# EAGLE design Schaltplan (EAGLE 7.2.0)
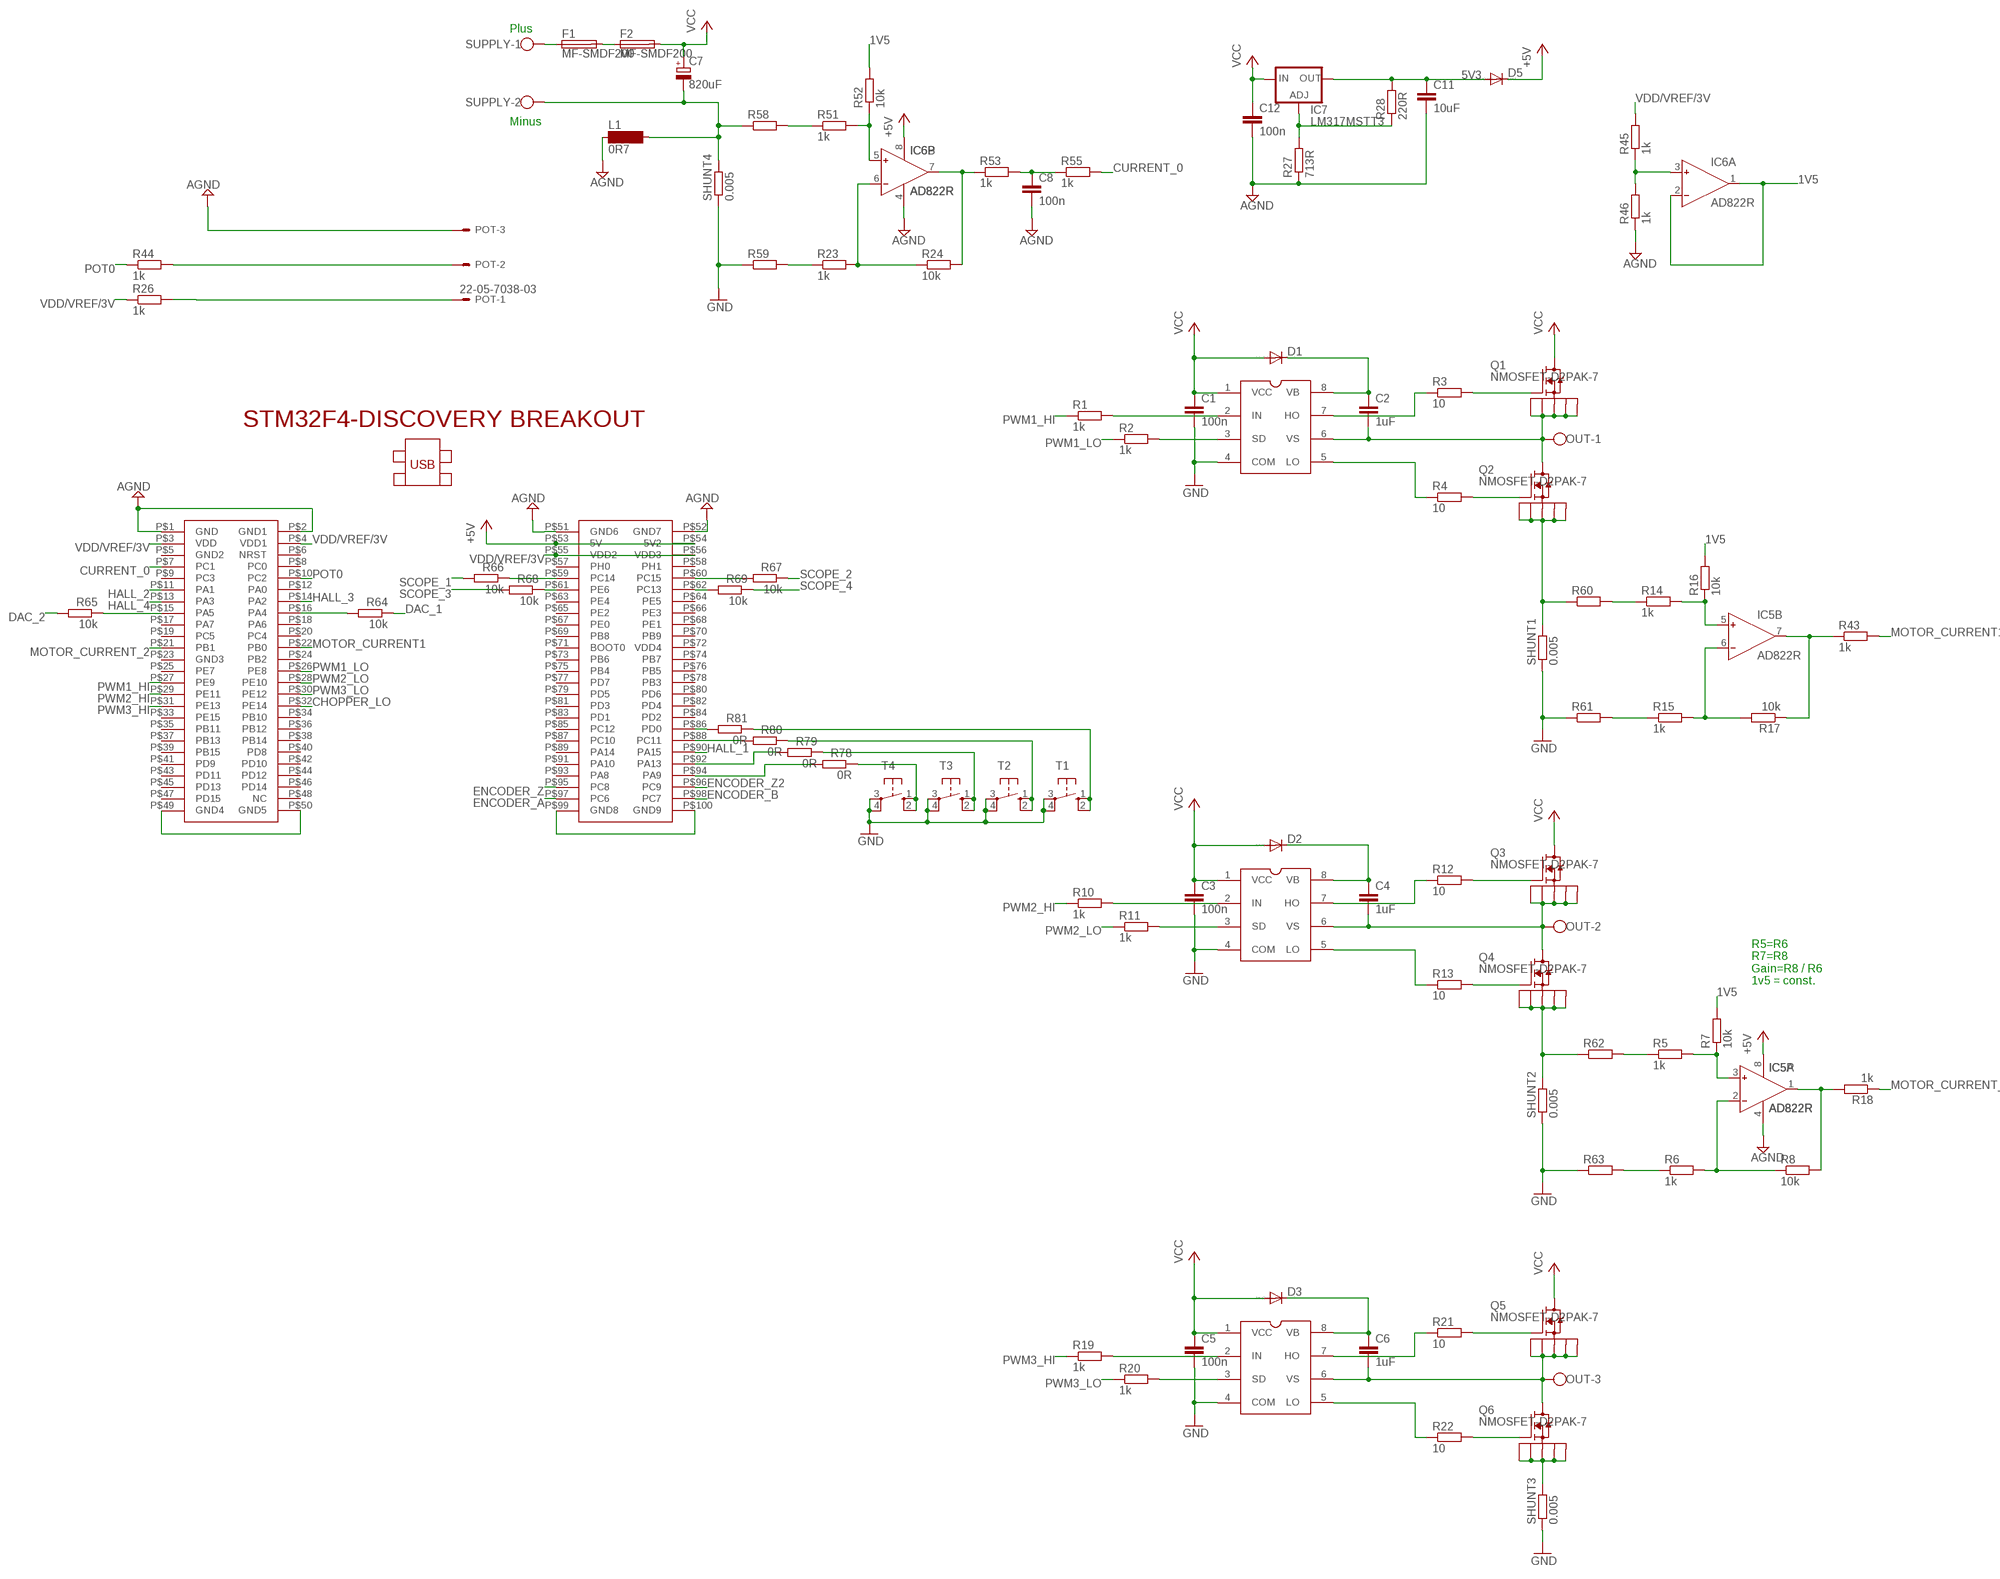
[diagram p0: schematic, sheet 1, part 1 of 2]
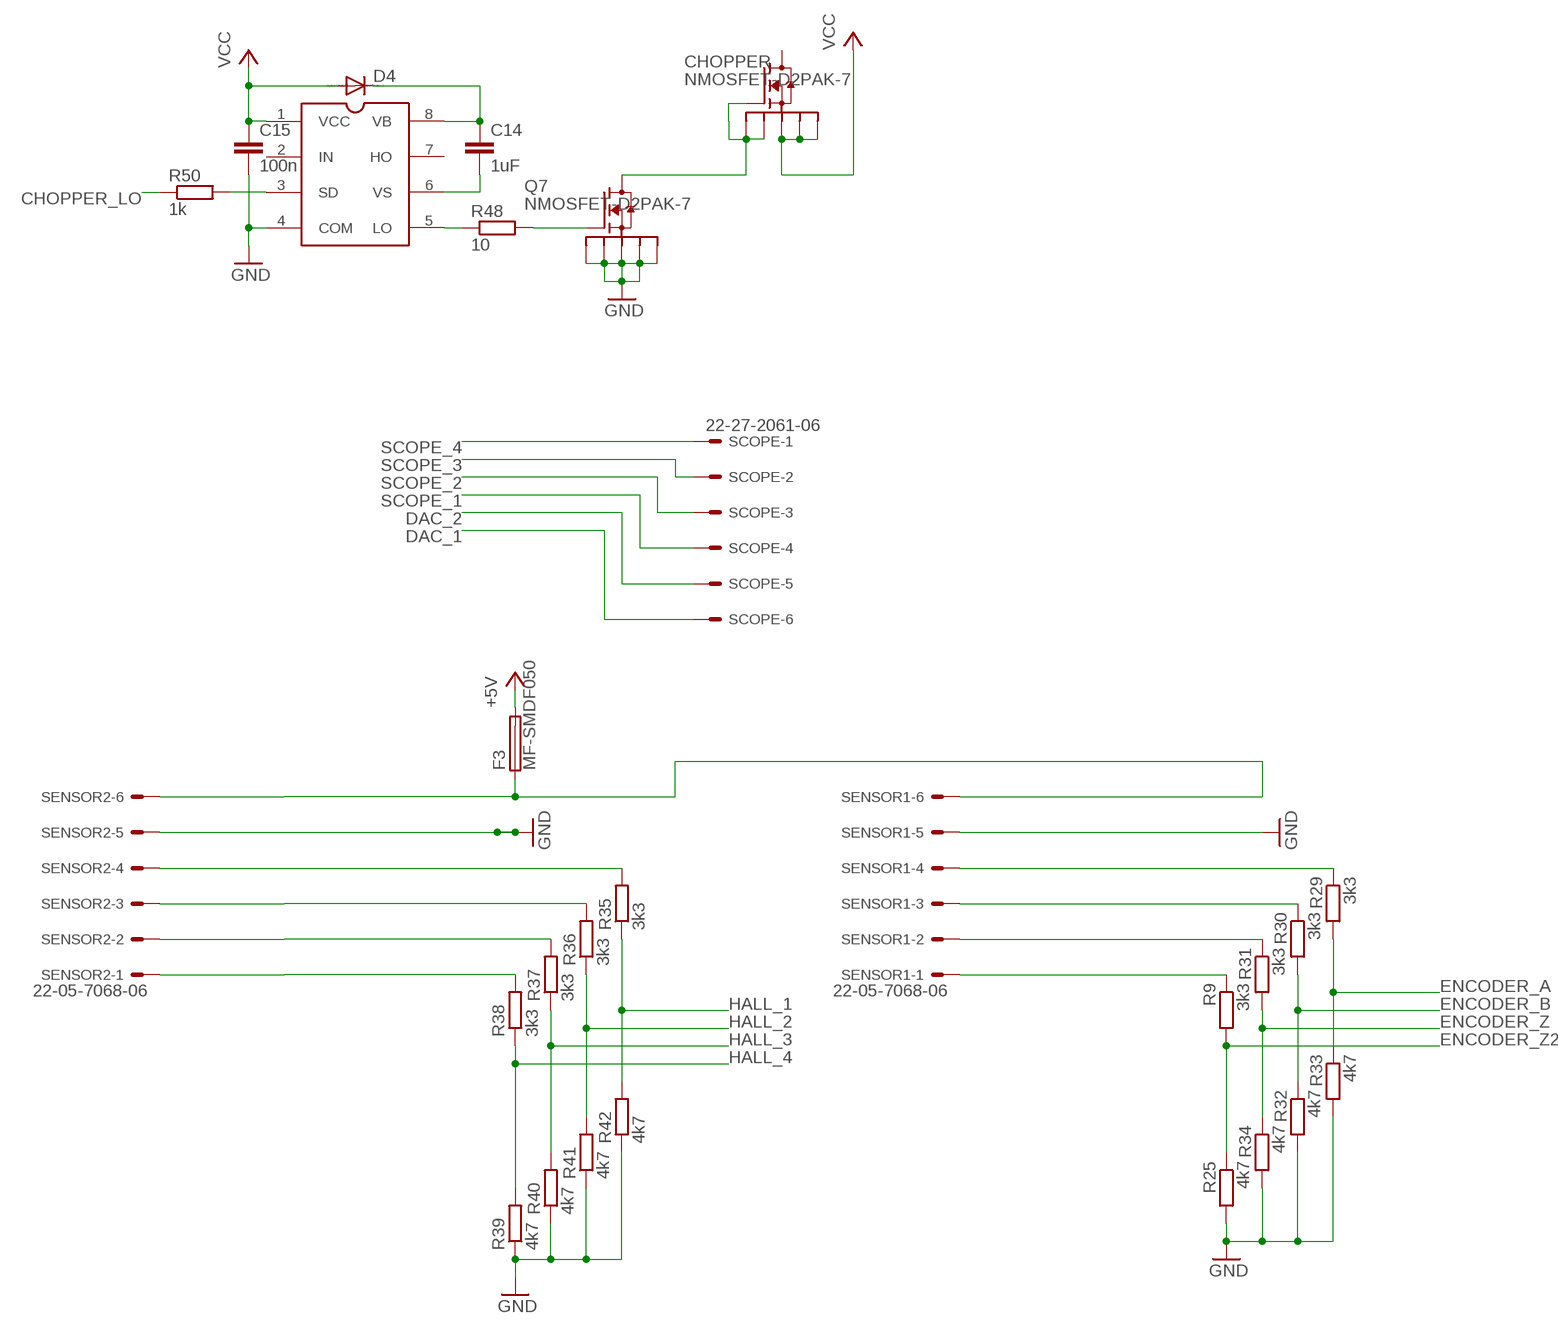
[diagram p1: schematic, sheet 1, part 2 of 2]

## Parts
C1  100n  C-EUC0805K  [C0805K]
C2  1uF  C-EUC0805K  [C0805K]
C3  100n  C-EUC0805K  [C0805K]
C4  1uF  C-EUC0805K  [C0805K]
C5  100n  C-EUC0805K  [C0805K]
C6  1uF  C-EUC0805K  [C0805K]
C7  820uF  CPOL-EUE7.5-18  [E7,5-18]
C8  100n  C-EUC0805K  [C0805K]
C11  10uF  C-EUC0805K  [C0805K]
C12  100n  C-EUC0805K  [C0805K]
C14  1uF  C-EUC0805K  [C0805K]
C15  100n  C-EUC0805K  [C0805K]
CHOPPER  NMOSFET-D2PAK-7  [D2PAK-7]
D1  DIODE-DO214AC  [DO214AC]
D2  DIODE-DO214AC  [DO214AC]
D3  DIODE-DO214AC  [DO214AC]
D4  DIODE-DO214AC  [DO214AC]
D5  DIODE-DO214AC  [DO214AC]
F1  MF-SMDF200  [MF-SMDF050]
F2  MF-SMDF200  [MF-SMDF050]
F3  MF-SMDF050  [MF-SMDF050]
IC1  IR2104S  [IR2104S]
IC2  IR2104S  [IR2104S]
IC3  IR2104S  [IR2104S]
IC4  IR2104S  [IR2104S]
IC5  AD822R  [SO8]
IC6  AD822R  [SO8]
IC7  LM317MSTT3  [SOT223]
L1  0R7  SM-1206  [SM-1206]
OUT  W237-103  [W237-103]
POT  22-05-7038-03  [7395-03]
Q1  NMOSFET-D2PAK-7  [D2PAK-7]
Q2  NMOSFET-D2PAK-7  [D2PAK-7]
Q3  NMOSFET-D2PAK-7  [D2PAK-7]
Q4  NMOSFET-D2PAK-7  [D2PAK-7]
Q5  NMOSFET-D2PAK-7  [D2PAK-7]
Q6  NMOSFET-D2PAK-7  [D2PAK-7]
Q7  NMOSFET-D2PAK-7  [D2PAK-7]
R1  1k  R-EU_M0805  [M0805]
R2  1k  R-EU_M0805  [M0805]
R3  10  R-EU_M0805  [M0805]
R4  10  R-EU_M0805  [M0805]
R5  1k  R-EU_M0805  [M0805]
R6  1k  R-EU_M0805  [M0805]
R7  10k  R-EU_M0805  [M0805]
R8  10k  R-EU_M0805  [M0805]
R9  3k3  R-EU_M0805  [M0805]
R10  1k  R-EU_M0805  [M0805]
R11  1k  R-EU_M0805  [M0805]
R12  10  R-EU_M0805  [M0805]
R13  10  R-EU_M0805  [M0805]
R14  1k  R-EU_M0805  [M0805]
R15  1k  R-EU_M0805  [M0805]
R16  10k  R-EU_M0805  [M0805]
R17  10k  R-EU_M0805  [M0805]
R18  1k  R-EU_M0805  [M0805]
R19  1k  R-EU_M0805  [M0805]
R20  1k  R-EU_M0805  [M0805]
R21  10  R-EU_M0805  [M0805]
R22  10  R-EU_M0805  [M0805]
R23  1k  R-EU_M0805  [M0805]
R24  10k  R-EU_M0805  [M0805]
R25  4k7  R-EU_M0805  [M0805]
R26  1k  R-EU_M0805  [M0805]
R27  713R  R-EU_M0805  [M0805]
R28  220R  R-EU_M0805  [M0805]
R29  3k3  R-EU_M0805  [M0805]
R30  3k3  R-EU_M0805  [M0805]
R31  3k3  R-EU_M0805  [M0805]
R32  4k7  R-EU_M0805  [M0805]
R33  4k7  R-EU_M0805  [M0805]
R34  4k7  R-EU_M0805  [M0805]
R35  3k3  R-EU_M0805  [M0805]
R36  3k3  R-EU_M0805  [M0805]
R37  3k3  R-EU_M0805  [M0805]
R38  3k3  R-EU_M0805  [M0805]
R39  4k7  R-EU_M0805  [M0805]
R40  4k7  R-EU_M0805  [M0805]
R41  4k7  R-EU_M0805  [M0805]
R42  4k7  R-EU_M0805  [M0805]
R43  1k  R-EU_M0805  [M0805]
R44  1k  R-EU_M0805  [M0805]
R45  1k  R-EU_M0805  [M0805]
R46  1k  R-EU_M0805  [M0805]
R48  10  R-EU_M0805  [M0805]
R50  1k  R-EU_M0805  [M0805]
R51  1k  R-EU_M0805  [M0805]
R52  10k  R-EU_M0805  [M0805]
R53  1k  R-EU_M0805  [M0805]
R55  1k  R-EU_M0805  [M0805]
R58  R-EU_M0805  [M0805]
R59  R-EU_M0805  [M0805]
R60  R-EU_M0805  [M0805]
R61  R-EU_M0805  [M0805]
R62  R-EU_M0805  [M0805]
R63  R-EU_M0805  [M0805]
R64  10k  R-EU_M0805  [M0805]
R65  10k  R-EU_M0805  [M0805]
R66  10k  R-EU_M0805  [M0805]
R67  10k  R-EU_M0805  [M0805]
R68  10k  R-EU_M0805  [M0805]
R69  10k  R-EU_M0805  [M0805]
R78  0R  R-EU_M0805  [M0805]
R79  0R  R-EU_M0805  [M0805]
R80  0R  R-EU_M0805  [M0805]
R81  0R  R-EU_M0805  [M0805]
SCOPE  22-27-2061-06  [6410-06]
SENSOR1  22-05-7068-06  [7395-06]
SENSOR2  22-05-7068-06  [7395-06]
SHUNT1  0.005  R-EU_R2512  [R2512]
SHUNT2  0.005  R-EU_R2512  [R2512]
SHUNT3  0.005  R-EU_R2512  [R2512]
SHUNT4  0.005  R-EU_R2512  [R2512]
SUPPLY  W237-102  [W237-102]
T1  10-XX  [B3F-10XX]
T2  10-XX  [B3F-10XX]
T3  10-XX  [B3F-10XX]
T4  10-XX  [B3F-10XX]
U$1  STM32F4-DISCOVERY  [STM32F4-DISCOVERY]

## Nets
1: C2.2 IC1.6(VS) OUT.1 Q1.S1 Q1.S2 Q1.S3 Q1.S4 Q1.S5 Q2.D
1V5: IC6.1(A:OUT) IC6.2(A:IN-) R7.2 R16.2 R52.2
2: C4.2 IC2.6(VS) OUT.2 Q3.S1 Q3.S2 Q3.S3 Q3.S4 Q3.S5 Q4.D
3 [power]: C6.2 IC3.6(VS) OUT.3 Q5.S1 Q5.S2 Q5.S3 Q5.S4 Q5.S5 Q6.D
5V3: C11.1 D5.A IC7.4(OUT) R28.2
+5V: D5.C F3.2 IC5.8(P:V+) IC6.8(P:V+) U$1.P$53(5V) U$1.P$54(5V2)
AGND: C8.2 C11.2 C12.2 IC5.4(P:V-) IC6.4(P:V-) L1.1 POT.3 R27.1 R46.1 U$1.P$1(GND) U$1.P$2(GND1) U$1.P$51(GND6) U$1.P$52(GND7)
CHOPPER_LO: R50.1 U$1.P$32(PE14)
CURRENT_0: R55.2 U$1.P$7(PC1)
DAC_1: R64.1 SCOPE.6
DAC_2: R65.2 SCOPE.5
ENCODER_A: R29.2 R33.1 U$1.P$97(PC6)
ENCODER_B: R30.2 R32.1 U$1.P$98(PC7)
ENCODER_Z: R31.2 R34.1 U$1.P$95(PC8)
ENCODER_Z2: R9.2 R25.1 U$1.P$96(PC9)
GND [power]: C1.2 C3.2 C5.2 C15.2 IC1.4(COM) IC2.4(COM) IC3.4(COM) IC4.4(COM) Q7.S1 Q7.S2 Q7.S3 Q7.S4 Q7.S5 R25.2 R32.2 R33.2 R34.2 R39.1 R40.1 R41.1 R42.1 R59.1 R61.1 R63.1 SENSOR1.5 SENSOR2.5 SHUNT1.1 SHUNT2.1 SHUNT3.1 SHUNT4.1 T1.3(P) T1.4(P1) T2.3(P) T2.4(P1) T3.3(P) T3.4(P1) T4.3(P) T4.4(P1)
HALL_1: R35.1 R42.2 U$1.P$90(PA15)
HALL_2: R36.1 R41.2 U$1.P$11(PA1)
HALL_3: R37.1 R40.2 U$1.P$14(PA2)
HALL_4: R38.1 R39.2 U$1.P$13(PA3)
MOTOR_CURRENT1: R43.2 U$1.P$22(PB0)
MOTOR_CURRENT_2: R18.1 U$1.P$21(PB1)
N$1: IC1.7(HO) R3.1
N$2: Q1.G R3.2
N$3: Q2.G R4.2
N$4: IC1.5(LO) R4.1
N$5: C2.1 D1.C IC1.8(VB)
N$6: IC2.7(HO) R12.1
N$7: IC5.2(A:IN-) R6.2 R8.1
N$8: IC1.2(IN) R1.2
N$9: IC1.3(SD) R2.2
N$10: Q3.G R12.2
N$11: Q2.S1 Q2.S2 Q2.S3 Q2.S4 Q2.S5 R60.1 SHUNT1.2
N$12: IC5.3(A:IN+) R5.2 R7.1
N$13: IC5.1(A:OUT) R8.2 R18.2
N$14: Q4.G R13.2
N$15: IC2.5(LO) R13.1
N$16: C4.1 D2.C IC2.8(VB)
N$17: IC2.2(IN) R10.2
N$18: IC2.3(SD) R11.2
N$19: Q4.S1 Q4.S2 Q4.S3 Q4.S4 Q4.S5 R62.1 SHUNT2.2
N$20: IC5.5(B:IN+) R14.2 R16.1
N$21: IC5.6(B:IN-) R15.2 R17.2
N$22: IC5.7(B:OUT) R17.1 R43.1
N$23: IC3.7(HO) R21.1
N$24: Q5.G R21.2
N$25: Q6.G R22.2
N$26: IC3.5(LO) R22.1
N$27: C6.1 D3.C IC3.8(VB)
N$28: IC3.2(IN) R19.2
N$29: IC3.3(SD) R20.2
N$30: R23.1 R59.2
N$31: F3.1 SENSOR1.6 SENSOR2.6
N$32: IC6.3(A:IN+) R45.1 R46.2
N$33: IC7.1(ADJ) R27.2 R28.1
N$34: R29.1 SENSOR1.4
N$35: R30.1 SENSOR1.3
N$36: C8.1 R53.2 R55.1
N$37: R31.1 SENSOR1.2
N$38: R64.2 U$1.P$16(PA4)
N$39: R65.1 U$1.P$15(PA5)
N$40: R79.2 U$1.P$92(PA13)
N$41: R9.1 SENSOR1.1
N$42: R35.2 SENSOR2.4
N$43: R36.2 SENSOR2.3
N$44: R37.2 SENSOR2.2
N$45: R38.2 SENSOR2.1
N$46: R66.1 U$1.P$59(PC14)
N$47: R68.1 U$1.P$61(PE6)
N$48: R69.2 U$1.P$62(PC13)
N$49: R67.2 U$1.P$60(PC15)
N$50: POT.1 R26.2
N$51: R80.2 U$1.P$88(PC11)
N$52: R81.2 U$1.P$86(PD0)
N$53: CHOPPER.G CHOPPER.S1 CHOPPER.S2 Q7.D
N$54: R51.1 R58.2
N$55: R78.1 T4.1(S) T4.2(S1)
N$56: R5.1 R62.2
N$57: POT.2 R44.2
N$58: R78.2 U$1.P$94(PA9)
N$59: R79.1 T3.1(S) T3.2(S1)
N$62 [power]: F1.1 SUPPLY.1
N$63 [power]: C7.- L1.2 R58.1 SHUNT4.2 SUPPLY.2
N$64: R80.1 T2.1(S) T2.2(S1)
N$68: R6.1 R63.2
N$71: Q7.G R48.2
N$72: IC6.6(B:IN-) R23.2 R24.1
N$73: C14.1 D4.C IC4.8(VB)
N$74: C14.2 IC4.6(VS)
N$75: IC4.5(LO) R48.1
N$77: IC4.3(SD) R50.2
N$79: IC6.7(B:OUT) R24.2 R53.1
N$80: IC6.5(B:IN+) R51.2 R52.1
N$83: F1.2 F2.1
N$84: R81.1 T1.1(S) T1.2(S1)
N$85: R14.1 R60.2
N$86: R15.1 R61.2
N$89: Q6.S1 Q6.S2 Q6.S3 Q6.S4 Q6.S5 SHUNT3.2
N$91: U$1.P$99(GND8) U$1.P$100(GND9)
N$92: U$1.P$49(GND4) U$1.P$50(GND5)
POT0: R44.1 U$1.P$10(PC2)
PWM1_HI: R1.1 U$1.P$27(PE9)
PWM1_LO: R2.1 U$1.P$26(PE8)
PWM2_HI: R10.1 U$1.P$29(PE11)
PWM2_LO: R11.1 U$1.P$28(PE10)
PWM3_HI: R19.1 U$1.P$31(PE13)
PWM3_LO: R20.1 U$1.P$30(PE12)
SCOPE_1: R66.2 SCOPE.4
SCOPE_2: R67.1 SCOPE.3
SCOPE_3: R68.2 SCOPE.2
SCOPE_4: R69.1 SCOPE.1
VCC [power]: C1.1 C3.1 C5.1 C7.+ C12.1 C15.1 CHOPPER.S3 CHOPPER.S4 CHOPPER.S5 D1.A D2.A D3.A D4.A F2.2 IC1.1(VCC) IC2.1(VCC) IC3.1(VCC) IC4.1(VCC) IC7.3(IN) Q1.D Q3.D Q5.D
VDD/VREF/3V: R26.1 R45.2 U$1.P$3(VDD) U$1.P$4(VDD1) U$1.P$55(VDD2) U$1.P$56(VDD3)
Unconnected: CHOPPER.D IC4.2(IN) IC4.7(HO) U$1.P$5(GND2) U$1.P$6(NRST) U$1.P$8(PC0) U$1.P$9(PC3) U$1.P$12(PA0) U$1.P$17(PA7) U$1.P$18(PA6) U$1.P$19(PC5) U$1.P$20(PC4) U$1.P$23(GND3) U$1.P$24(PB2) U$1.P$25(PE7) U$1.P$33(PE15) U$1.P$34(PB10) U$1.P$35(PB11) U$1.P$36(PB12) U$1.P$37(PB13) U$1.P$38(PB14) U$1.P$39(PB15) U$1.P$40(PD8) U$1.P$41(PD9) U$1.P$42(PD10) U$1.P$43(PD11) U$1.P$44(PD12) U$1.P$45(PD13) U$1.P$46(PD14) U$1.P$47(PD15) U$1.P$48(NC) U$1.P$57(PH0) U$1.P$58(PH1) U$1.P$63(PE4) U$1.P$64(PE5) U$1.P$65(PE2) U$1.P$66(PE3) U$1.P$67(PE0) U$1.P$68(PE1) U$1.P$69(PB8) U$1.P$70(PB9) U$1.P$71(BOOT0) U$1.P$72(VDD4) U$1.P$73(PB6) U$1.P$74(PB7) U$1.P$75(PB4) U$1.P$76(PB5) U$1.P$77(PD7) U$1.P$78(PB3) U$1.P$79(PD5) U$1.P$80(PD6) U$1.P$81(PD3) U$1.P$82(PD4) U$1.P$83(PD1) U$1.P$84(PD2) U$1.P$85(PC12) U$1.P$87(PC10) U$1.P$89(PA14) U$1.P$91(PA10) U$1.P$93(PA8)

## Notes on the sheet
- Plus
- Minus
- R5=R6
  R7=R8
  Gain=R8 / R6
  1v5 = const.

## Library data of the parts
C1-C6 C8 C11 C12 C14 C15 = rcl:C-EU: CAPACITOR, European symbol
C7 = rcl:CPOL-EU: POLARIZED CAPACITOR, European symbol
CHOPPER Q1-Q7 = D2PAK-7:NMOSFET-D2PAK-7
D1-D5 = diode:DIODE-: DIODE
F1-F3 = fuse:MF-SMDF: MF-SMDF Series - PRC Resettable Fuses
IC1-IC4 = ir-2104:IR2104S: Half Bridge Mosfet - IGBT driver SOIC
IC5 IC6 = analog-devices:AD822: Single-Supply, Rail-to-Rail Low Power FET-Input Op Amp Source: http://www.analog.com/static/imported-files/data_sheets/AD822.pdf; MF: ANALOG DEVICES; MPN: AD822BRZ; OC_FARNELL: 1651303
IC7 = v-reg:LM317?*: 500 mA Adjustable Output Positive Voltage Regulator Source: http://www.onsemi.co.jp .. LM317M-D.PDF
L1 = inductor-neosid:SM-1206: INDUCTOR; OC_FARNELL: unknown; OC_NEWARK: unknown
OUT = con-wago-500:W237-103: WAGO SCREW CLAMP; MPN: 237-103; OC_FARNELL: unknown; OC_NEWARK: 18M7116
POT = con-molex:22-?-03: CONNECTOR wire to board 2.54 mm (.1 inch) pitch header; OC_FARNELL: unknown; OC_NEWARK: unknown
R1-R5 R7-R46 R48 R50-R53 R55 R64-R69 R78-R81 = resistor:R-EU_: RESISTOR, European symbol
R6 R58-R63 SHUNT1-SHUNT4 = rcl:R-EU_: RESISTOR, European symbol
SCOPE SENSOR1 SENSOR2 = con-molex:22-?-06: CONNECTOR wire to board 2.54 mm (.1 inch) pitch header; OC_FARNELL: unknown; OC_NEWARK: unknown
SUPPLY = con-wago-500:W237-102: WAGO SCREW CLAMP; MPN: 237-102; OC_FARNELL: unknown; OC_NEWARK: 70K9898
T1-T4 = switch-omron:10-XX: OMRON SWITCH; MPN: B3F-1000; OC_FARNELL: 176432; OC_NEWARK: 36M3542
U$1 = STM32F4-DISCOVERY:STM32F4-DISCOVERY

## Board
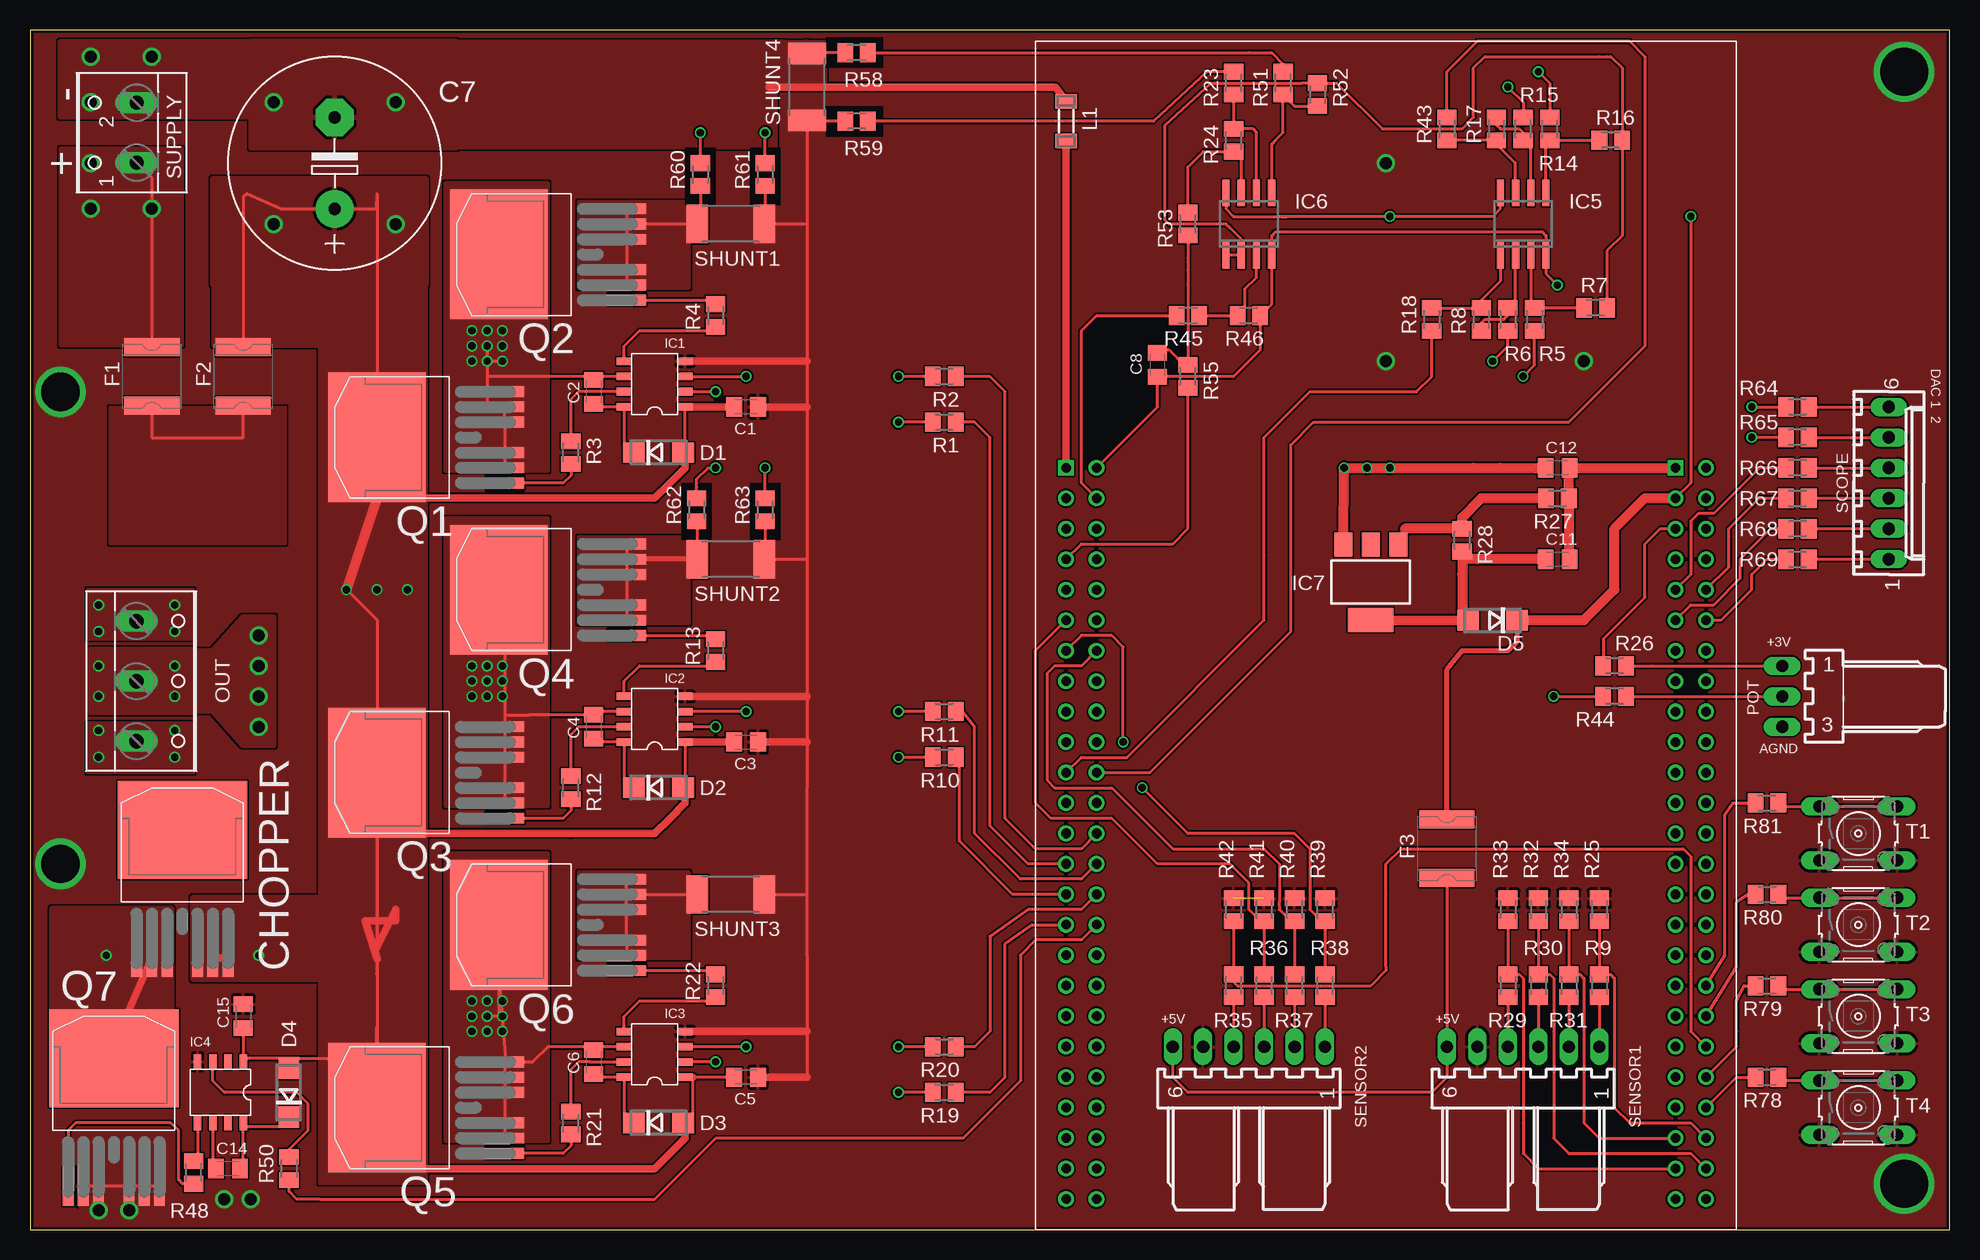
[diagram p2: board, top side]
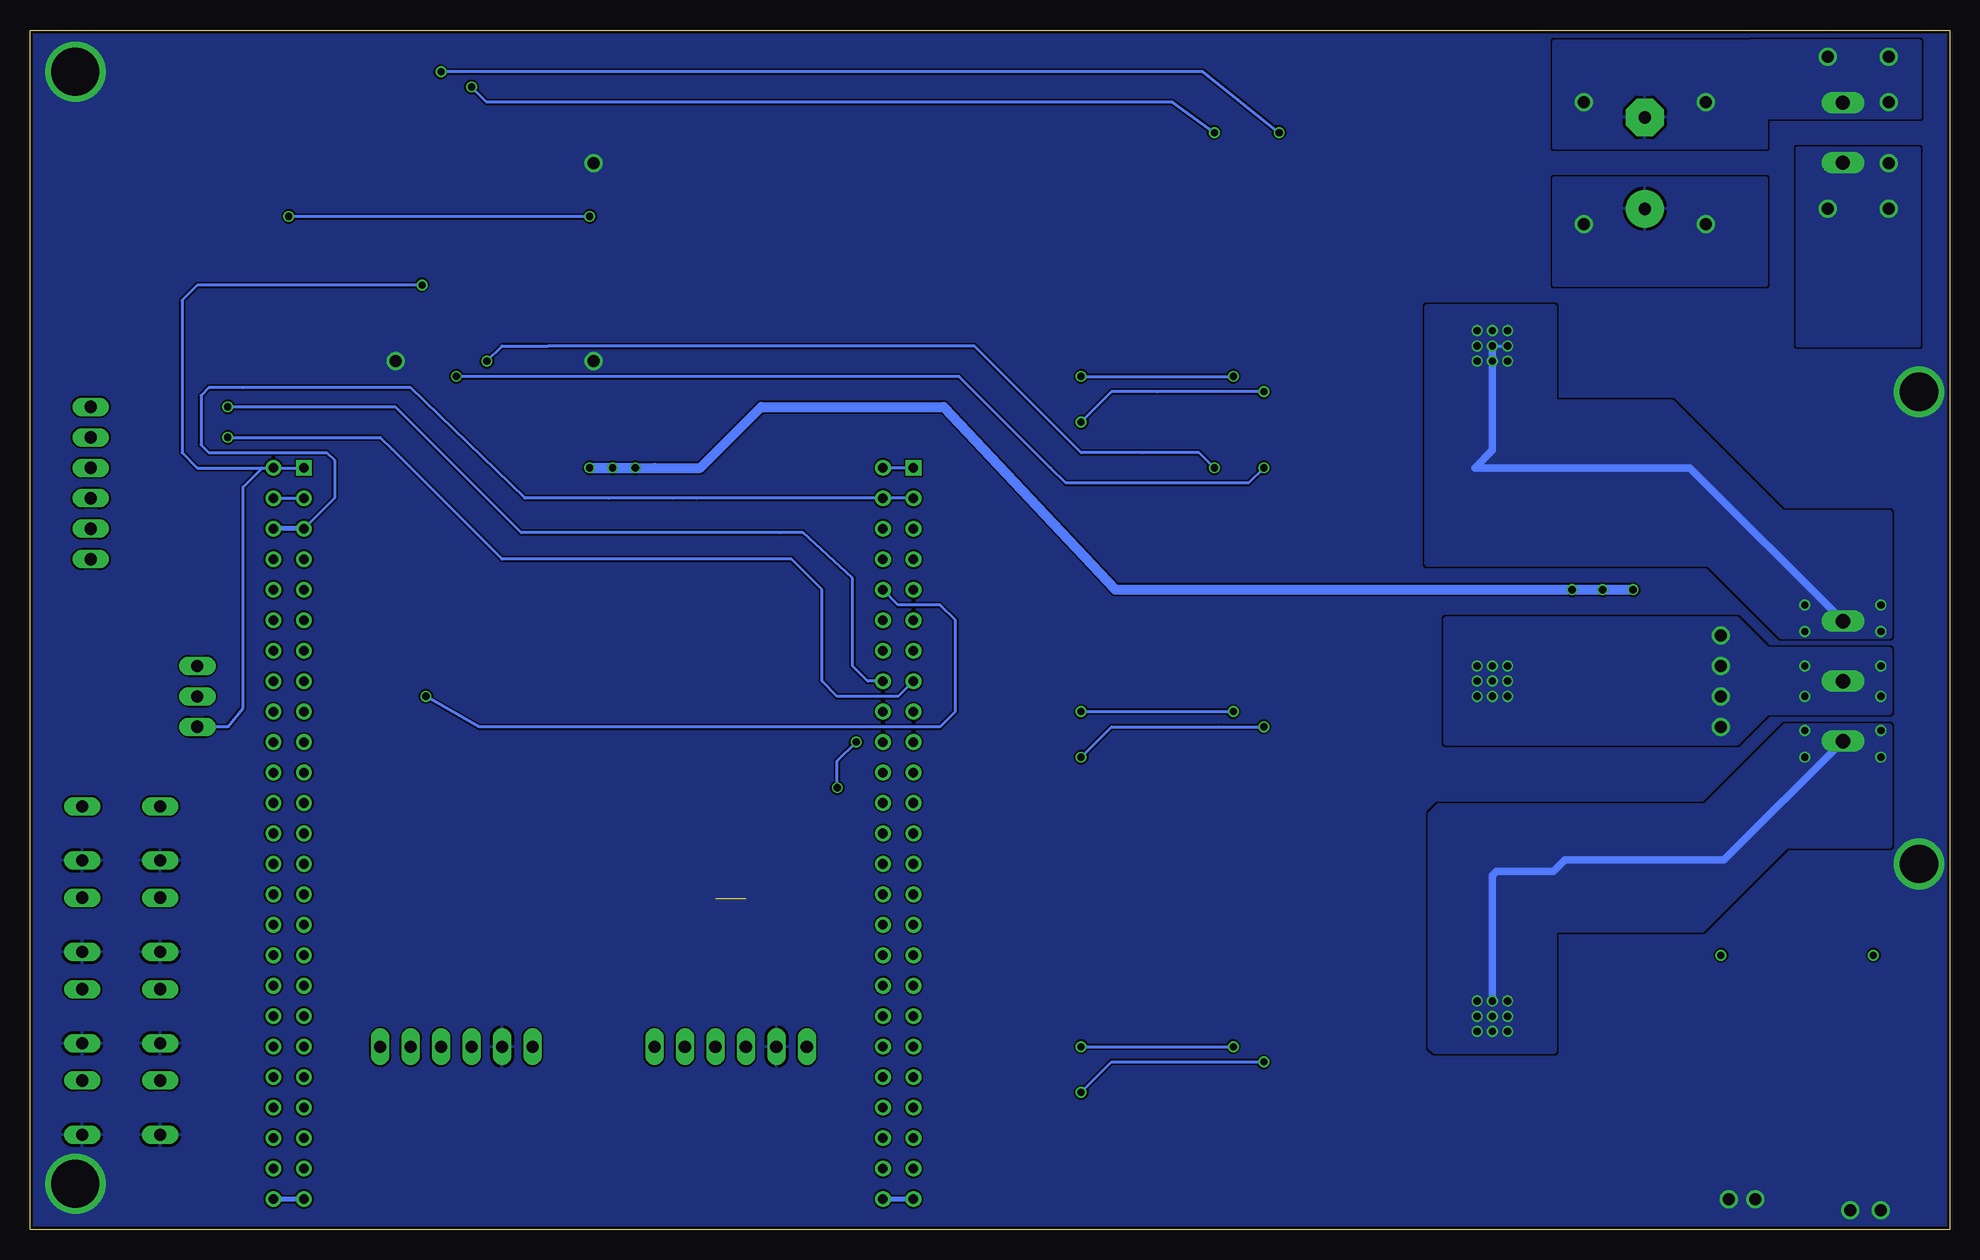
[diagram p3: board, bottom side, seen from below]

Size 160 x 100 mm. Coordinates in mm from the lower left corner, seen from the top.
Outline: 0,0 160,0 160,100 0,100 0,0
Copper layers (1*16): Top 0.035mm / dielectric 1.5mm / Bottom 0.035mm
Design rules "Elecrow_2-layer_eagle_rule": minimum track width 6mil, minimum drill 12mil, track to track 6mil, track to pad 6mil, pad to pad 6mil, via to via 6mil, smd to smd 0mil, copper to edge 10mil, drill to drill 10mil, minimum pad ring 10mil, minimum via ring 6mil, stop-mask expansion 2mil, vias tented up to drill 100mil, thermal gap 10mil

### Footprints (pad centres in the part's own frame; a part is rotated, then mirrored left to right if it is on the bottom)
C0805K = smd 1.3 x 1.6: 1 -1,0; 2 1,0
E7,5-18 = drill 1.016 pad 3.15: + -3.81,0 | drill 1.016 pad 3.15 octagon: - 3.81,0
D2PAK-7 = smd 10.8 x 8.15: D 0,4.1 | smd 0.9 x 3.2: G -3.81,-6.56; S1 -2.54,-6.56; S2 -1.27,-6.56; S3 1.27,-6.56; S4 2.54,-6.56; S5 3.81,-6.56
DO214AC = smd 1.8 x 1.7: A 2.05,0; C -2.05,0
MF-SMDF050 = smd 1.5 x 4.6: 1 -2.45,0; 2 2.45,0
IR2104S = smd 1.27 x 0.635: 1 0,3.81; 2 0,2.54; 3 0,1.27; 4 0,0; 5 5.08,0; 6 5.08,1.27; 7 5.08,2.54; 8 5.08,3.81
SO8 = smd 0.6 x 2.2: 1 -1.905,-2.6; 2 -0.635,-2.6; 3 0.635,-2.6; 4 1.905,-2.6; 5 1.905,2.6; 6 0.635,2.6; 7 -0.635,2.6; 8 -1.905,2.6
SOT223 = smd 1.5 x 2: 1 -2.3,-3.15; 2 0,-3.15; 3 2.3,-3.15 | smd 3.8 x 2: 4 0,3.15
SM-1206 = smd 1.2 x 1.8: 1 -1.65,0; 2 1.65,0
W237-103 = drill 1.194 long: 1 -5,-1.29; 2 0,-1.29; 3 5,-1.29
7395-03 = drill 1.016 long: 1 2.54,0; 2 0,0; 3 -2.54,0
M0805 = smd 1.3 x 1.6: 1 -0.95,0; 2 0.95,0
6410-06 = drill 1.016 long: 1 6.35,0; 2 3.81,0; 3 1.27,0; 4 -1.27,0; 5 -3.81,0; 6 -6.35,0
7395-06 = drill 1.016 long: 1 6.35,0; 2 3.81,0; 3 1.27,0; 4 -1.27,0; 5 -3.81,0; 6 -6.35,0
R2512 = smd 1.8 x 3.2: 1 -2.8,0; 2 2.8,0
W237-102 = drill 1.194 long: 1 -2.5,-1.27; 2 2.5,-1.27
B3F-10XX = drill 1.016 long: 1 -3.251,2.261; 2 3.251,2.261; 3 -3.251,-2.261; 4 3.251,-2.261
STM32F4-DISCOVERY = drill 0.8 square: P$1 -27.94,30.48; P$51 22.86,30.48 | drill 0.8: P$2 -25.4,30.48; P$3 -27.94,27.94; P$4 -25.4,27.94; P$5 -27.94,25.4; P$6 -25.4,25.4; P$7 -27.94,22.86; P$8 -25.4,22.86; P$9 -27.94,20.32; P$10 -25.4,20.32; P$11 -27.94,17.78; P$12 -25.4,17.78; P$13 -27.94,15.24; P$14 -25.4,15.24; P$15 -27.94,12.7; P$16 -25.4,12.7; P$17 -27.94,10.16; P$18 -25.4,10.16; P$19 -27.94,7.62; P$20 -25.4,7.62; P$21 -27.94,5.08; P$22 -25.4,5.08; P$23 -27.94,2.54; P$24 -25.4,2.54; P$25 -27.94,0; P$26 -25.4,0; P$27 -27.94,-2.54; P$28 -25.4,-2.54; P$29 -27.94,-5.08; P$30 -25.4,-5.08; P$31 -27.94,-7.62; P$32 -25.4,-7.62; P$33 -27.94,-10.16; P$34 -25.4,-10.16; P$35 -27.94,-12.7; P$36 -25.4,-12.7; P$37 -27.94,-15.24; P$38 -25.4,-15.24; P$39 -27.94,-17.78; P$40 -25.4,-17.78; P$41 -27.94,-20.32; P$42 -25.4,-20.32; P$43 -27.94,-22.86; P$44 -25.4,-22.86; P$45 -27.94,-25.4; P$46 -25.4,-25.4; P$47 -27.94,-27.94; P$48 -25.4,-27.94; P$49 -27.94,-30.48; P$50 -25.4,-30.48; P$52 25.4,30.48; P$53 22.86,27.94; P$54 25.4,27.94; P$55 22.86,25.4; P$56 25.4,25.4; P$57 22.86,22.86; P$58 25.4,22.86; P$59 22.86,20.32; P$60 25.4,20.32; P$61 22.86,17.78; P$62 25.4,17.78; P$63 22.86,15.24; P$64 25.4,15.24; P$65 22.86,12.7; P$66 25.4,12.7; P$67 22.86,10.16; P$68 25.4,10.16; P$69 22.86,7.62; P$70 25.4,7.62; P$71 22.86,5.08; P$72 25.4,5.08; P$73 22.86,2.54; P$74 25.4,2.54; P$75 22.86,0; P$76 25.4,0; P$77 22.86,-2.54; P$78 25.4,-2.54; P$79 22.86,-5.08; P$80 25.4,-5.08; P$81 22.86,-7.62; P$82 25.4,-7.62; P$83 22.86,-10.16; P$84 25.4,-10.16; P$85 22.86,-12.7; P$86 25.4,-12.7; P$87 22.86,-15.24; P$88 25.4,-15.24; P$89 22.86,-17.78; P$90 25.4,-17.78; P$91 22.86,-20.32; P$92 25.4,-20.32; P$93 22.86,-22.86; P$94 25.4,-22.86; P$95 22.86,-25.4; P$96 25.4,-25.4; P$97 22.86,-27.94; P$98 25.4,-27.94; P$99 22.86,-30.48; P$100 25.4,-30.48

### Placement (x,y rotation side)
C1  59.69,68.58 0 top
C2  46.99,69.85 90 top
C3  59.69,40.64 0 top
C4  46.99,41.91 90 top
C5  59.69,12.7 0 top
C6  46.99,13.97 90 top
C7  25.4,88.9 90 top
C8  93.98,72.07 270 top
C11  127.32,55.88 0 top
C12  127.32,63.5 0 top
C14  16.51,5.08 180 top
C15  17.78,17.78 90 top
CHOPPER  12.7,29.21 0 top
D1  52.39,64.77 0 top
D2  52.39,36.83 0 top
D3  52.39,8.89 0 top
D4  21.59,11.43 90 top
D5  121.92,50.8 180 top
F1  10.16,71.12 270 top
F2  17.78,71.12 90 top
F3  118.11,31.75 90 top
IC1  54.61,72.39 180 top
IC2  54.61,44.45 180 top
IC3  54.61,16.51 180 top
IC4  13.97,13.97 270 top
IC5  124.46,83.82 0 top
IC6  101.6,83.82 0 top
IC7  111.76,53.98 180 top
L1  86.36,92.39 90 top
OUT  10.16,45.72 270 top
POT  146.05,44.45 90 top
Q1  33.02,66.04 90 top
Q2  43.18,81.28 90 top
Q3  33.02,38.1 90 top
Q4  43.18,53.34 90 top
Q5  33.02,10.16 90 top
Q6  43.18,25.4 90 top
Q7  6.99,10.16 0 top
R1  76.2,67.31 180 top
R2  76.2,71.12 180 top
R3  45.09,64.77 270 top
R4  57.15,76.2 90 top
R5  125.41,75.88 90 top
R6  123.19,75.88 90 top
R7  130.49,76.83 0 top
R8  120.97,75.88 90 top
R9  130.81,20.32 90 top
R10  76.2,39.37 180 top
R11  76.2,43.18 180 top
R12  45.09,36.83 270 top
R13  57.15,48.26 90 top
R14  126.68,91.76 270 top
R15  124.46,91.76 270 top
R16  131.76,90.81 0 top
R17  122.24,91.76 90 top
R18  116.84,75.88 90 top
R19  76.2,11.43 180 top
R20  76.2,15.24 180 top
R21  45.09,8.89 270 top
R22  57.15,20.32 90 top
R23  100.33,95.57 270 top
R24  100.33,90.81 270 top
R25  130.81,26.67 90 top
R26  132.08,46.99 0 top
R27  127.32,60.96 180 top
R28  119.38,57.47 270 top
R29  123.19,20.32 90 top
R30  125.73,20.32 90 top
R31  128.27,20.32 90 top
R32  125.73,26.67 90 top
R33  123.19,26.67 90 top
R34  128.27,26.67 90 top
R35  100.33,20.32 270 top
R36  102.87,20.32 270 top
R37  105.41,20.32 270 top
R38  107.95,20.32 270 top
R39  107.95,26.67 270 top
R40  105.41,26.67 270 top
R41  102.87,26.67 270 top
R42  100.33,26.67 270 top
R43  118.11,91.76 90 top
R44  132.08,44.45 0 top
R45  96.52,76.2 180 top
R46  101.6,76.2 180 top
R48  13.65,4.76 270 top
R50  21.59,5.08 90 top
R51  104.46,95.57 270 top
R52  107.31,94.61 90 top
R53  96.52,83.82 270 top
R55  96.52,71.12 270 top
R58  68.9,98.11 0 top
R59  68.9,92.39 0 top
R60  55.88,87.95 90 top
R61  61.28,87.95 90 top
R62  55.56,60.01 90 top
R63  61.28,60.01 90 top
R64  147.32,68.58 180 top
R65  147.32,66.04 0 top
R66  147.32,63.5 0 top
R67  147.32,60.96 180 top
R68  147.32,58.42 0 top
R69  147.32,55.88 180 top
R78  144.78,12.7 180 top
R79  144.78,20.32 180 top
R80  144.78,27.94 180 top
R81  144.78,35.56 180 top
SCOPE  154.94,62.23 270 top
SENSOR1  124.46,15.24 0 top
SENSOR2  101.6,15.24 0 top
SHUNT1  58.42,83.82 180 top
SHUNT2  58.42,55.88 180 top
SHUNT3  58.42,27.94 180 top
SHUNT4  64.77,95.25 90 top
SUPPLY  7.62,91.44 90 top
T1  152.4,33.02 0 top
T2  152.4,25.4 0 top
T3  152.4,17.78 0 top
T4  152.4,10.16 0 top
U$1  114.3,33.02 0 top

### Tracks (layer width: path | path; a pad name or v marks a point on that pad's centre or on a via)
1  (via drill 0.6)
  Top 0.254: Q1.S4 Q1.S3 Q1.S2 Q1.S1 | 39.69,81.28 Q2.D | v38.1,73.66 v38.1,72.39 | v38.1,72.39 38.1,71.12 | 38.1,71.12 38.1,68.58 | v38.1,72.39 v39.37,72.39 | IC1.6 47.62,71.12 47.35,70.85 C2.2 46.72,71.12 38.1,71.12
  Bottom 0.254: v38.1,73.66 v36.83,73.66
  Bottom 0.61: OUT.1 21.65,63.5 Q1.S1 38.1,64.98 v38.1,72.39 v38.1,73.66
  other vias: 36.83,74.93 38.1,74.93 39.37,74.93 39.37,73.66 36.83,72.39 5.71,49.85 12.06,49.85 12.06,52.07 5.71,52.07
  pour Top (no thermals): 34.61,87.31 43.18,87.31 43.18,63.18 34.61,63.18
  pour Bottom (isolate 0.406, no thermals): 20,55.56 43.5,55.56 43.5,76.83 33.02,76.83 33.02,68.9 23.18,68.9 13.97,59.69 5.08,59.69 5.08,49.53 13.97,49.53
  pour Top (isolate 0.406, no thermals): 4.76,49.21 13.65,49.21 13.65,53.34 4.76,53.34
1V5
  Top 0.254: R7.2 131.44,81.59 132.72,82.87 R16.2 132.71,96.84 131.76,97.79 131.44,97.79 130.81,97.79 121.28,97.79 120.33,96.84 120.33,92.71 119.38,91.76 113.03,91.76 112.71,91.76 108.9,95.57 R52.2 106.68,95.57 106.05,95.57 101.92,95.57 98.74,95.57 | 98.42,95.57 98.74,95.57 | 98.42,95.57 94.61,92.08 94.61,84.14 94.93,83.82 99.69,83.82 100.01,83.5 100.97,82.55 IC6.2 IC6.1 | 98.42,95.57 98.74,95.57
2  (via drill 0.6, 1)
  Top 0.254: Q3.S1 Q3.S2 Q3.S3 Q3.S4 Q3.S5 39.58,42.86 | Q4.D 39.58,52.84 39.58,42.86 | IC2.6 47.26,43.18 C4.2 41.64,42.91 41.59,42.86 39.58,42.86
  other vias: 36.83,45.72 36.83,46.99 38.1,46.99 39.37,46.99 36.83,44.45 38.1,44.45 39.37,44.45 39.37,45.72 5.71,44.45 5.71,46.99 12.06,46.99 12.06,44.45 38.1,45.72 19.05,41.91 19.05,44.45 19.05,46.99 19.05,49.53
  pour Top (no thermals): 34.61,59.37 43.18,59.37 43.18,35.24 34.61,35.24
  pour Bottom (isolate 0.406, no thermals): 41.91,50.8 17.78,50.8 15.24,48.26 5.08,48.26 5.08,43.18 15.24,43.18 17.78,40.64 41.91,40.64
  pour Top (isolate 0.406, no thermals): 5.08,48.26 13.65,48.26 13.65,43.18 5.08,43.18
  pour Top (no thermals): 13.34,48.26 15.24,48.26 17.78,51.12 20.32,51.12 20.32,40.32 17.78,40.32 15.24,43.18 13.34,43.18
3  (via drill 0.6)
  Top 0.254: Q5.S5 Q5.S4 Q5.S3 Q5.S2 Q5.S1 | Q5.S5 39.05,13.65 39.69,13.97 39.05,21.91 | Q6.D 39.05,25.37 39.05,21.91 | 39.05,21.91 39.05,17.78 v38.1,17.78 | C6.2 47.62,15.24 IC3.6 43.18,15.24 41.91,13.97 Q5.S5 | 39.05,21.91 39.05,25.4 39.37,25.4 | 39.37,25.4 38.73,25.4 39.05,25.72 39.37,25.4
  Bottom 0.61: OUT.3 18.79,30.8 32.07,30.8 33.02,29.84 37.78,29.84 38.1,29.53 v38.1,19.05
  other vias: 36.83,16.51 36.83,19.05 36.83,17.78 39.37,19.05 39.37,16.51 39.37,17.78 38.1,16.51 5.71,39.37 5.71,41.59 12.06,41.59 12.06,39.37
  pour Top (no thermals): 34.61,31.43 43.18,31.43 43.18,7.3 34.61,7.3
  pour Bottom (isolate 0.406, no thermals): 5.08,41.91 13.65,41.91 20.32,35.24 42.55,35.24 43.18,34.61 43.18,15.24 42.86,14.92 33.02,14.92 33.02,24.77 33.34,25.08 20.64,25.08 13.65,32.07 5.08,32.07
  pour Top (isolate 0.406, no thermals): 4.76,38.1 13.65,38.1 13.65,42.23 4.76,42.23
5V3
  Top 0.254: 119.38,51.29 D5.A 119.84,50.77 | R28.2 119.38,55.88
  Top 0.813: IC7.4 119.84,50.77 | 119.38,51.29 119.38,54.61 119.38,55.88 120.65,55.88 C11.1
+5V  (via drill 0.6)
  Top 0.254: IC6.8 99.69,85.09 100.33,84.45 104.14,84.45 | 104.14,84.45 104.78,84.45 | 122.56,87 IC5.8 122.56,85.09 121.92,84.45 | 121.92,84.45 v113.35,84.45 | v113.35,84.45 104.14,84.45 | 121.92,84.45 v113.35,84.45 | v138.43,84.45 138.43,83.19 138.43,62.23 U$1.P$53
  Top 0.406: F3.2 118.11,46.67 119.38,48.26 123.19,48.26 123.97,49.04 D5.C
  Top 0.813: D5.C 129.54,50.8 132.08,53.34 132.08,58.42 134.62,60.96 U$1.P$53
  Bottom 0.254: v113.35,84.45 v138.43,84.45 | U$1.P$54 U$1.P$53
AGND  (via drill 0.6)
  Top 0.254: 128.27,55.93 C11.2 | 128.27,63.45 C12.2 | U$1.P$2 93.98,68.58 C8.2 94.57,71.07 94.61,71.12 94.93,71.12 100.33,71.12 102.55,73.34 R46.1 103.5,77.16 IC6.4 103.5,82.87 103.82,83.19 126.05,83.19 126.36,82.87 IC5.4 126.36,79.69 v127.32,78.74
  Top 0.61: L1.1 86.36,78.04 U$1.P$1
  Top 0.813: 128.27,55.93 R27.1 128.27,63.45 | C12.2 U$1.P$51
  Bottom 0.254: U$1.P$52 140.65,63.5 142.24,61.91 142.24,43.5 143.51,41.91 POT.3 | U$1.P$52 U$1.P$51 | U$1.P$1 U$1.P$2 | v127.32,78.74 144.78,78.74 146.05,78.74 147.32,77.47 147.32,64.77 146.05,63.5 U$1.P$52
CHOPPER_LO
  Top 0.254: U$1.P$32 87.63,24.13 83.82,24.13 82.55,22.86 82.55,12.38 77.79,7.62 57.15,7.62 52.07,2.54 24.13,2.54 22.23,2.54 21.59,3.17 R50.1
CURRENT_0
  Top 0.254: U$1.P$7 87.63,57.15 95.25,57.15 96.52,58.42 R55.2
DAC_1
  Top 0.254: R64.1 SCOPE.6
DAC_2
  Top 0.254: R65.2 SCOPE.5
ENCODER_A
  Top 0.254: R29.2 122.87,21.27 R29.2 | R29.2 124.14,21.27 124.46,20.95 124.46,8.89 124.46,6.35 125.73,5.08 U$1.P$97 | R33.1 R29.2
ENCODER_B
  Top 0.254: 126.36,21.27 R30.2 R32.1 | 126.36,21.27 | 126.36,21.27 | 126.36,21.27 126.68,21.27 127,20.95 127,16.51 127,7.62 128.27,6.35 138.43,6.35 U$1.P$98
ENCODER_Z
  Top 0.254: U$1.P$95 130.81,7.62 129.54,8.89 129.54,20.95 129.22,21.27 R31.2 R34.1
ENCODER_Z2
  Top 0.254: U$1.P$96 138.43,8.89 133.35,8.89 132.08,10.16 132.08,20.95 131.76,21.27 R9.2 R25.1
GND  (via drill 1, 3.2 pad 0.25, 4 pad 0.25)  (1 unrouted)
  Top 0.254: SHUNT4.1 64.77,90.81 | 64.77,90.81 64.77,83.82 | 64.77,83.82 64.77,72.39 64.77,68.58 64.77,55.88 | 64.77,55.88 64.77,44.45 64.77,40.64 64.77,39.69 64.77,38.1 64.77,36.83 64.77,36.2 64.77,27.94 | 64.77,12.7 64.77,14.92 64.77,16.51 | SHUNT3.1 64.77,27.94 | SHUNT4.1 64.77,90.81 | 64.77,90.81 64.77,88.9 | 64.77,83.82 SHUNT1.1 61.22,84.83 61.28,84.89 R61.1 | 64.77,16.51 64.77,22.86 64.77,27.94 | Q7.S5 Q7.S4 Q7.S3 Q7.S2 Q7.S1 | 64.77,55.88 SHUNT2.1 61.22,56.89 61.28,56.95 R63.1 | SHUNT4.1 65.46,92.45 65.72,92.71 66.04,92.39 R59.1 | 64.77,92.71 64.77,90.81 | IC3.4 64.77,16.51
  Top 0.61: IC2.4 64.77,44.45 | IC1.4 64.77,72.39 | IC3.4 64.77,16.51 | C5.2 64.77,12.7 | C3.2 64.77,40.64 | C1.2 64.77,68.58
  other vias: 129.54,72.39 5.71,1.59 8.26,1.59 16.19,2.54 18.41,2.54 113.03,88.9 113.03,72.39 2.54,30.48 2.54,69.85 156.21,3.81 156.21,96.52
  pour Top (no thermals): 66.36,93.66 66.36,91.12 62.87,91.12 62.87,93.66
  pour Top (no thermals): 60.01,85.41 62.55,85.41 62.55,81.92 60.01,81.92
  pour Top (no thermals): 60.01,57.47 62.55,57.47 62.55,53.98 60.01,53.98
  pour Top (no thermals): 60.01,30.16 62.55,30.16 62.55,26.04 60.01,26.04
  pour Top (no thermals): 4.13,5.4 4.13,1.59 11.75,1.59 11.75,5.4
  pour Top (rank 4): 0,100 160,100 160,0 0,0
  pour Bottom (rank 4): 0,100 160,100 160,0 0,0
HALL_1
  Top 0.254: U$1.P$90 138.43,16.51 138.43,21.27 138.43,31.11 137.79,31.75 114.3,31.75 113.03,30.48 113.03,27.94 113.03,21.91 113.03,21.59 111.76,20.32 100.65,20.32 100.33,20.64 R35.1 R42.2
HALL_2
  Top 0.254: U$1.P$11 83.82,48.26 83.82,35.56 85.09,34.29 90.17,34.29 91.44,33.02 93.98,30.48 99.38,30.48 100.01,30.48 101.6,28.89 101.6,26.67 102.87,25.4 | R41.2 103.5,25.4 102.87,25.4 | 102.87,25.4 R36.1
HALL_3
  Top 0.254: U$1.P$14 87.63,46.99 86.36,46.99 85.72,46.99 85.41,46.99 84.77,46.35 84.77,37.47 85.41,36.83 90.17,36.83 91.44,35.56 93.98,33.02 95.25,31.75 102.87,31.75 104.14,30.48 104.14,27.3 104.14,26.99 104.14,26.67 105.09,25.72 R40.2 R37.1
HALL_4  (via drill 0.6)
  Top 0.254: v92.71,36.83 93.98,35.56 96.52,33.02 105.41,33.02 106.68,31.75 106.68,26.67 107.63,25.72 R39.2 R38.1 | v91.12,40.64 91.12,48.58 90.17,49.53 87.63,49.53 U$1.P$13
  Bottom 0.254: v92.71,36.83 92.71,39.05 v91.12,40.64
MOTOR_CURRENT1
  Top 0.254: U$1.P$22 93.34,38.1 105.09,49.85 105.09,65.41 107,67.31 107.31,67.31 107.63,67.31 128.27,67.31 134.62,73.66 134.62,82.87 134.62,97.79 133.35,99.06 120.97,99.06 120.65,99.06 120.33,98.74 118.11,96.52 R43.2
MOTOR_CURRENT_2
  Top 0.254: U$1.P$21 87.63,39.37 91.44,39.37 102.87,50.8 102.87,56.2 102.87,66.04 106.68,69.85 115.57,69.85 116.84,71.12 116.84,73.98 | 116.84,73.34 116.84,73.98 | 116.84,73.98 R18.1
N$1
  Top 0.254: IC1.7 45.72,69.85 45.09,69.22 45.09,68.9 45.09,68.58 R3.1
N$2
  Top 0.254: R3.2 45.09,62.87 44.45,62.23 Q1.G
N$3
  Top 0.254: R4.2 56.52,77.47 52.07,77.47 Q2.G
N$4
  Top 0.254: IC1.5 49.53,73.66 50.8,74.93 56.83,74.93 R4.1
N$5
  Top 0.254: D1.C 50.16,64.77 49.53,65.41 IC1.8 47.31,68.58 47.04,68.85 C2.1
N$6
  Top 0.254: IC2.7 45.72,41.91 45.09,41.27 45.09,40.96 45.09,40.64 R12.1
N$7
  Top 0.254: IC5.2 123.83,77.47 R6.2 123.19,76.2 122.87,75.88 121.28,75.88 120.97,75.56 R8.1
N$8  (via drill 0.6)
  Top 0.254: R1.2 v72.39,67.31 | IC1.2 v57.15,69.85
  Bottom 0.254: v57.15,69.85 66.04,69.85 69.85,69.85 | 69.85,69.85 v72.39,67.31 69.85,69.85
N$9  (via drill 0.6)
  Top 0.254: R2.2 v72.39,71.12 | IC1.3 v59.69,71.12
  Bottom 0.254: v72.39,71.12 v59.69,71.12
N$10
  Top 0.254: R12.2 45.09,34.92 44.45,34.29 Q3.G
N$11
  Top 0.254: Q2.S5 Q2.S4 | Q2.S4 Q2.S3 | Q2.S3 Q2.S2 | Q2.S2 Q2.S1 Q2.S2 | Q2.S4 Q2.S3 | Q2.S4 SHUNT1.2 55.88,84.08 R60.1
  Top 0.406: SHUNT1.2 55.88,83.82 | 55.88,83.82 SHUNT1.2 | SHUNT1.2 55.88,83.82
  pour Top (isolate 0.406, no thermals): 45.72,85.72 54.93,85.72 54.93,78.42 45.72,78.42
  pour Top (no thermals): 54.29,85.41 54.93,85.09 54.29,85.09
N$12
  Top 0.254: 125.09,77.15 R5.2 | IC5.3 125.09,77.47 125.41,77.15 R5.2 | R7.1 R5.2
N$13
  Top 0.254: IC5.1 122.56,79.06 120.97,77.47 R8.2 R18.2
N$14
  Top 0.254: Q4.G 50.06,49.21 50.38,49.53 56.83,49.53 56.84,49.21 R13.2
N$15
  Top 0.254: IC2.5 49.53,45.72 50.8,46.99 56.83,46.99 R13.1
N$16
  Top 0.254: D2.C 49.85,36.83 49.53,37.15 IC2.8 47.26,40.64 C4.1
N$17  (via drill 0.6)
  Top 0.254: R10.2 v72.39,39.37 | v57.15,41.91 IC2.2
  Bottom 0.254: v72.39,39.37 69.85,41.91 60.96,41.91 v57.15,41.91
N$18  (via drill 0.6)
  Top 0.254: R11.2 v72.39,43.18 | v59.69,43.18 IC2.3
  Bottom 0.254: v72.39,43.18 v59.69,43.18
N$19
  Top 0.254: Q4.S5 Q4.S4 Q4.S3 Q4.S2 Q4.S1 | 55.88,55.88 SHUNT2.2 55.62,59.06 R62.1
  Top 0.406: SHUNT2.2 50.8,55.88 Q4.S4
  pour Top (isolate 0.406, no thermals): 45.72,57.78 54.93,57.78 54.93,50.48 45.72,50.48
N$20
  Top 0.254: IC5.5 126.36,90.17 126.68,90.49 | 126.68,90.49 R14.2 R16.1 | 126.68,90.49 126.69,90.48
N$21
  Top 0.254: IC5.6 125.09,90.49 124.78,90.81 R15.2 124.46,91.44 124.14,91.76 123.83,91.76 122.56,91.76 122.24,92.08 R17.2
N$22
  Top 0.254: IC5.7 123.83,88.9 122.24,90.49 R17.1 R43.1
N$23
  Top 0.254: IC3.7 46.67,13.97 45.72,13.97 45.09,13.34 45.09,13.02 R21.1
N$24
  Top 0.254: R21.2 45.09,6.99 44.45,6.35 Q5.G
N$25
  Top 0.254: Q6.G 50.8,21.59 56.83,21.59 56.84,21.27 R22.2
N$26
  Top 0.254: IC3.5 49.53,17.78 50.8,19.05 56.52,19.05 R22.1
N$27
  Top 0.254: D3.C 49.85,9.53 49.53,9.21 IC3.8 47.62,12.7 C6.1
N$28  (via drill 0.6)
  Top 0.254: R19.2 v72.39,11.43 | v57.15,13.97 IC3.2
  Bottom 0.254: v72.39,11.43 69.85,13.97 v57.15,13.97
N$29  (via drill 0.6)
  Top 0.254: R20.2 v72.39,15.24 | v59.69,15.24 IC3.3
  Bottom 0.254: v72.39,15.24 v59.69,15.24
N$30
  Top 0.254: R23.1 98.11,96.52 93.66,92.39 R59.2
N$31
  Top 0.254: F3.1 118.11,17.78 118.11,16.51 SENSOR1.6 118.11,12.7 116.84,11.43 96.52,11.43 95.25,12.7 SENSOR2.6
N$32
  Top 0.254: R45.1 R46.2 101.28,76.83 101.28,78.42 102.23,79.38 IC6.3
N$33
  Top 0.254: R27.2 | IC7.1 113.98,57.78 114.62,58.42
  Top 0.813: R27.2 120.97,60.96 119.38,59.37 R28.1 114.62,58.42
N$34
  Top 0.254: R29.1 SENSOR1.4
N$35
  Top 0.254: 125.89,19.85 126.05,20 126.05,19.69 R30.1 SENSOR1.3
N$36
  Top 0.254: R53.2 96.52,80.96 96.52,80.64 96.52,80.01 96.52,78.74 R55.1 96.2,72.07 94.93,73.34 94.25,73.34 C8.1
N$37
  Top 0.254: R31.1 SENSOR1.2
N$38  (via drill 0.6)
  Top 0.254: v143.51,68.58 R64.2
  Bottom 0.254: U$1.P$16 90.17,45.72 91.44,46.99 91.44,54.29 95.57,58.1 97.47,58.1 119.06,58.1 129.54,68.58 131.13,68.58 v143.51,68.58
N$39  (via drill 0.6)
  Top 0.254: R65.1 v143.51,66.04
  Bottom 0.254: U$1.P$15 87.63,44.45 92.71,44.45 93.98,45.72 93.98,53.34 96.52,55.88 120.65,55.88 129.86,65.09 130.81,66.04 v143.51,66.04
N$40
  Top 0.254: U$1.P$92 142.24,15.24 142.24,16.51 142.24,19.05 142.88,20.32 R79.2
N$41
  Top 0.254: R9.1 SENSOR1.1
N$42
  Top 0.254: 100.17,19.53 R35.2 SENSOR2.4
N$43
  Top 0.254: R36.2 SENSOR2.3
N$44
  Top 0.254: R37.2 SENSOR2.2
N$45
  Top 0.254: R38.2 SENSOR2.1
N$46
  Top 0.254: R66.1 144.15,63.5 140.34,59.69 139.06,59.69 138.43,59.05 138.43,54.61 U$1.P$59
N$47
  Top 0.254: U$1.P$61 138.43,52.07 140.34,52.07 142.56,54.29 142.56,55.88 145.1,58.42 R68.1
N$48
  Top 0.254: U$1.P$62 140.97,50.8 143.51,53.34 143.51,54.61 144.78,55.88 R69.2
N$49
  Top 0.254: U$1.P$60 141.6,55.24 141.6,56.52 141.6,57.78 141.6,58.42 144.15,60.96 R67.2
N$50
  Top 0.254: 135.25,46.99 R26.2 POT.1
N$51
  Top 0.254: U$1.P$88 141.29,20.32 142.24,21.91 142.24,27.3 143.19,27.94 R80.2
N$52
  Top 0.254: U$1.P$86 141.29,22.86 141.29,34.61 141.92,35.56 R81.2
N$53  (via drill 0.6)
  Top 0.61: 7.62,16.8 CHOPPER.S1
  other vias: 6.35,22.86
  pour Top (isolate 0.406, no thermals): 11.75,26.67 11.75,15.24 1.91,15.24 1.91,26.67
N$54
  Top 0.254: R58.2 101.6,98.11 103.5,98.11 104.46,97.16 R51.1
N$55
  Top 0.254: R78.1 146.01,12.42 T4.1 T4.2
N$56  (via drill 0.6)
  Top 0.254: v124.46,71.12 125.41,72.07 R5.1 | R62.2 55.56,61.91 55.56,62.23 55.56,62.55 56.52,63.5 v57.15,63.5
  Bottom 0.254: v57.15,63.5 58.42,62.23 73.66,62.23 74.93,63.5 82.55,71.12 v124.46,71.12
N$57
  Top 0.254: R44.2 POT.2
N$58
  Top 0.254: U$1.P$94 142.24,12.7 R78.2
N$59
  Top 0.254: R79.1 146.01,20.04 T3.1 T3.2
N$62  (via drill 1)
  Top 0.254: SUPPLY.1 10.16,87.67 v10.16,85.09 F1.1
  other vias: 5.08,85.09 5.08,88.9
  pour Top (no thermals): 12.7,73.66 2.54,73.66 2.54,90.17 12.7,90.17
  pour Bottom (no thermals): 2.54,73.66 12.7,73.66 12.7,90.17 2.54,90.17
N$63  (via drill 1)
  Top 0.254: R58.1 64.83,98.11 SHUNT4.2
  Top 0.61: L1.2 85.47,95.25 61.59,95.25 | 64.39,98.05 SHUNT4.2
  other vias: 5.08,97.79 10.16,97.79 5.08,93.98 20.32,93.98 30.48,93.98
  pour Top: 33.02,99.06 33.02,90.17 62.23,90.17 62.23,95.57 66.36,95.57 66.36,99.06
  pour Bottom (isolate 0.406): 15.24,90.17 15.24,99.06 33.02,99.06 33.02,90.17
  pour Bottom (no thermals): 2.54,99.06 2.54,92.71 16.51,92.71 16.51,99.06
  pour Top (no thermals): 18.41,99.06 18.41,92.71 2.54,92.71 2.54,99.06
  pour Top: 35.56,99.06 18.41,99.06 18.41,90.17 35.56,90.17
  pour Top (no thermals): 66.36,99.06 66.36,96.84 62.87,96.84 62.87,99.06
N$64
  Top 0.254: R80.1 146.01,27.66 T2.1 T2.2
N$68  (via drill 0.6)
  Top 0.254: R63.2 v61.28,63.5 | v121.92,72.39 123.19,73.66 R6.1
  Bottom 0.254: v121.92,72.39 120.65,73.66 116.84,73.66 81.28,73.66 72.39,64.77 67.31,64.77 62.55,64.77 v61.28,63.5
N$71
  Top 0.254: R48.2 12.7,3.81 12.38,4.13 12.38,8.26 11.75,8.89 3.81,8.89 3.17,8.26 Q7.G
N$72
  Top 0.254: R23.2 R24.1 101.92,91.75 102.23,91.44 IC6.6
N$73
  Top 0.254: D4.C 20.78,8.57 18.1,8.57 IC4.8 17.78,5.35 C14.1
N$74
  Top 0.254: IC4.6 15.24,5.71 15.51,5.45 C14.2
N$75
  Top 0.254: IC4.5 13.97,6.35 13.65,6.03 R48.1
N$77
  Top 0.254: R50.2 21.59,6.67 23.18,8.26 23.18,10.16 23.18,10.48 22.23,11.43 16.19,11.43 15.24,12.38 IC4.3
N$78
  cutout Top: 60.01,90.17 62.55,90.17 62.55,85.41 60.01,85.41
  cutout Top: 54.61,90.17 57.15,90.17 57.15,85.41 54.61,85.41
  cutout Top: 66.36,91.44 66.36,93.34 71.12,93.34 71.12,91.44
  cutout Top: 66.36,91.12 66.36,93.66 71.12,93.66 71.12,91.12
  cutout Top: 66.36,96.84 66.36,99.38 71.12,99.38 71.12,96.84
  cutout Top: 60.01,62.23 62.55,62.23 62.55,57.47 60.01,57.47
  cutout Top: 54.29,62.23 56.83,62.23 56.83,57.47 54.29,57.47
N$79
  Top 0.254: IC6.7 100.97,89.22 R24.2 | R24.2 | R53.1 96.52,88.58 97.79,89.86 R24.2
N$80
  Top 0.254: IC6.5 103.5,90.49 103.83,90.81 104.46,91.44 R51.2 105.41,93.67 R52.1
N$83
  Top 0.254: F1.2 10.16,66.04 17.78,66.04 F2.1
  pour Top (no thermals): 6.67,68.58 21.27,68.58 21.27,57.15 6.67,57.15
N$84
  Top 0.254: R81.1 146.01,35.28 T1.1 T1.2
N$85  (via drill 0.6)
  Top 0.254: R60.2 v55.88,91.44 | v125.73,96.52 126.68,95.57 R14.1
  Bottom 0.254: v55.88,91.44 62.23,96.52 v125.73,96.52
N$86  (via drill 0.6)
  Top 0.254: R61.2 v61.28,91.44 | v123.19,95.25 124.46,93.98 R15.1
  Bottom 0.254: v61.28,91.44 64.77,93.98 116.84,93.98 121.92,93.98 v123.19,95.25
N$89
  Top 0.254: Q6.S1 Q6.S2 Q6.S3 Q6.S4 | Q6.S4 Q6.S5 | Q6.S4 SHUNT3.2
  pour Top (isolate 0.406, no thermals): 45.72,29.84 54.93,29.84 54.93,22.54 45.72,22.54
N$91
  Bottom 0.406: U$1.P$99 U$1.P$100
N$92
  Bottom 0.406: U$1.P$49 U$1.P$50
POT0  (via drill 0.6)
  Top 0.254: v127,44.45 R44.1
  Bottom 0.254: U$1.P$10 87.63,52.07 84.14,52.07 82.87,50.8 82.87,43.18 84.14,41.91 122.56,41.91 v127,44.45
PWM1_HI
  Top 0.254: U$1.P$27 83.19,30.48 80.01,33.66 80.01,66.04 78.74,67.31 R1.1
PWM1_LO
  Top 0.254: R2.1 80.01,71.12 81.28,69.85 81.28,34.29 83.82,31.75 87.63,31.75 U$1.P$26
PWM2_HI
  Top 0.254: U$1.P$29 81.92,27.94 77.47,32.38 77.47,38.1 77.47,39.05 R10.1
PWM2_LO
  Top 0.254: U$1.P$28 87.63,29.21 82.55,29.21 78.74,33.02 78.74,41.91 77.47,43.5 R11.1
PWM3_HI
  Top 0.254: U$1.P$31 83.5,25.4 81.28,23.81 81.28,12.7 80.01,11.43 R19.1
PWM3_LO
  Top 0.254: U$1.P$30 87.63,26.67 83.19,26.67 80.01,24.45 80.01,16.51 78.74,15.24 R20.1
SCOPE_1
  Top 0.254: R66.2 SCOPE.4
SCOPE_2
  Top 0.254: R67.1 SCOPE.3
SCOPE_3
  Top 0.254: R68.2 SCOPE.2
SCOPE_4
  Top 0.254: R69.1 SCOPE.1
VCC  (via drill 0.6, 1)
  Top 0.254: 28.92,33.02 Q3.D 28.92,50.8 v26.38,53.34 28.92,60.96 Q1.D 28.92,86.07 | 28.92,33.02 28.92,22.54 Q5.D | Q5.D 28.9,14.29 | 28.9,14.29 28.89,16.83 | 30.48,5.08 28.89,5.08 28.89,5.4 28.92,5.42 Q5.D | 28.92,33.02 28.89,32.99 28.89,23.5 28.89,21.27 | C5.1 55.24,12.7 | C1.1 IC1.1 54.61,64.94 D1.A | 28.92,86.07 28.92,86.33 | 28.92,86.33 28.92,86.07 | 28.92,86.33 28.89,85.09 C7.+ 20.95,85.09 18.1,86.36 17.78,86.04 F2.2 | 28.92,86.33 28.92,86.07 | IC3.1 54.93,12.7 55.24,12.7 | 55.24,12.7 55.24,8.89 D3.A | IC2.1 54.61,37 D2.A | D4.A 20.78,14.29 18.1,14.29 IC4.1 C15.1 | D4.A 22.4,14.29 28.9,14.29 | 21.59,14.29 D4.A
  Top 0.406: v113.35,63.5 v111.44,63.5
  Top 0.61: 28.92,33.02 45.09,33.02 52.07,33.02 53.34,34.29 54.61,35.56 54.61,36.66 D2.A | 55.24,12.7 54.93,12.7 IC3.1 | C3.1 IC2.1 | C1.1 IC1.1 | 28.92,60.96 52.07,60.96 53.34,62.23 54.61,63.5 54.61,64.14 54.44,64.31 D1.A | 30.48,5.08 50.8,5.08 52.07,5.08 54.61,7.62 54.61,8.26 D3.A | CHOPPER.S4 CHOPPER.S5 | 28.89,23.5 30.48,26.67 30.48,25.72 27.94,25.72 28.92,22.54
  Top 0.813: IC7.3 v109.54,63.5 v111.44,63.5 v113.35,63.5 120.33,63.5 122.56,63.5 C12.1 | v26.38,53.34 28.92,60.96
  Bottom 0.813: v26.38,53.34 69.53,53.34 83.82,68.58 99.06,68.58 104.14,63.5 107.95,63.5 v109.54,63.5 | v109.54,63.5 v113.35,63.5 v109.54,63.5
  other vias: 31.46,53.34 28.92,53.34 20.32,83.82 30.48,83.82 19.05,22.86
  pour Top (no thermals): 33.02,80.01 33.02,3.81 24.13,3.81 24.13,80.01
  pour Top (no thermals): 15.24,73.66 24.13,73.66 24.13,80.01 15.24,80.01
  pour Top (isolate 0.406, rank 3, no thermals): 32.38,60.33 32.07,60.33 32.07,68.58
  pour Bottom (isolate 0.406): 15.24,87.63 33.02,87.63 33.02,78.74 15.24,78.74
  pour Top (isolate 0.406, no thermals): 13.65,27.62 24.77,27.62 25.08,23.81 25.08,20.95 13.65,20.95
  pour Top: 15.24,87.63 33.02,87.63 33.02,78.74 15.24,78.74
VDD/VREF/3V
  Top 0.254: R45.2 88.9,76.2 87.63,74.93 87.63,62.23 U$1.P$4 | U$1.P$55 135.89,58.42 134.62,57.15 134.62,52.7 132.72,50.8 132.08,50.16 131.13,49.22 R26.1
  Bottom 0.254: U$1.P$55 134.62,60.96 134.62,64.14 135.25,64.77 145.1,64.77 145.73,65.41 145.73,69.53 145.1,70.17 142.24,70.17 128.27,70.17 118.75,60.96 111.76,60.96 106.36,60.96 104.46,60.96 U$1.P$4 U$1.P$3
  Bottom 0.406: U$1.P$55 U$1.P$56

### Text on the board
tNames: - | + | DAC 1 2 | +3V | AGND | +5V | +5V
tRestrict: TOP
bRestrict: skycurveESC | rev1.0 | BOTTOM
